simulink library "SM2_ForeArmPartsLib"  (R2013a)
settings: Solver=ode45  StartTime=0.0  StopTime=10.0  RelTol=1e-3
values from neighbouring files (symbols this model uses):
  ID = ID(val==max(val))    [PD_NarrowRange.m]    (also in NyquistMinDist_v1.m = find(D==minDist,1))
  m = v*BEAM.rho    [FlexBeamModelConstruct2.m]    (also in FlexBeamModelConstruct3.m = BEAM.rho*v; FlexBeam_1D_Construct.m = REF.m/REF.l*a.*(linspace(1-OPT.MassBiais+1e-6,1+OPT.MassBiai; FlexBeam_3D_Construct.m = REF.m/REF.l*a.*(linspace(1-OPT.MassBiais+1e-6,1+OPT.MassBiai; FreeFlexBeam_3D_Construct.m = REF.m/REF.l*a.*tmp2)
  N = D(1)+(H4^2+H3^2)/H2^2-(E(1)*H4+F(1)*H3)/H2    [MGD.m]    (also in MGD2.m)
  s = -sign(imag(KGZ_fr_tmp))    [LinprogReguliOptimFunc_1.m]    (also in LinprogReguliOptimFunc_2.m; LinprogReguliOptimFunc_1 - Copie.m)
  X = cos(phi(i))*x+sin(phi(i))*y    [MGI.m]
  Y = fft(y(:,i),NFFT)/L    [fft_bis.m]    (also in MGI.m = -sin(phi(i))*x+cos(phi(i))*y)
  Z = z    [MGI.m]
undefined symbols (not defined in the file or in its folder): kg, rad, SimParam
libraries: sm_lib x48, SM2_ForeArmPartsLib x42

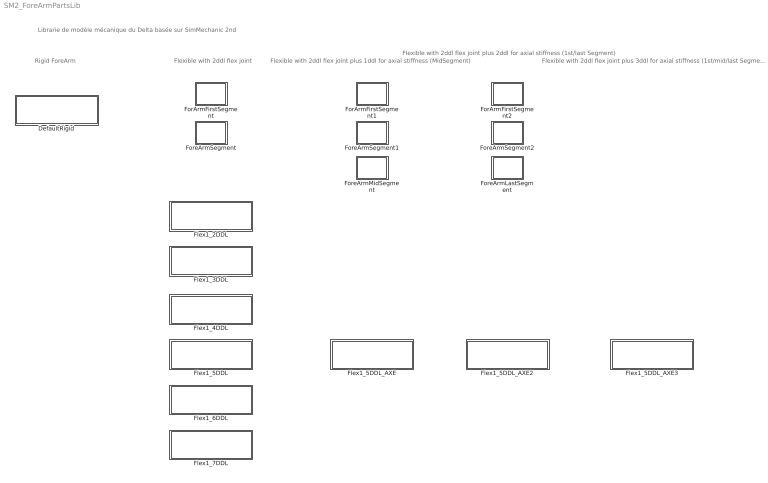
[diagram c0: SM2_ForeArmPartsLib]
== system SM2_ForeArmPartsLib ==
  note: Librarie de modèle mécanique du Delta basée sur SimMechanic 2nd
  note: Rigid ForeArm
  note: Flexible with 2ddl flex joint plus 1ddl for axial stiffness (MidSegment)
  note: Flexible with 2ddl flex joint
  note: Flexible with 2ddl flex joint plus 2ddl for axial stiffness (1st/last Segment)
  note: Flexible with 2ddl flex joint plus 3ddl for axial stiffness (1st/mid/last Segment)
  DefaultRigid : Subsystem  InitFcn=SimParam.ForeArm = RigidForeArm_paramInitFnc(RawParam,0);  VariantControl=foreArmVarDefault
  Flex1_2DDL : Subsystem  InitFcn=SimParam.ForeArm = flexPreCalcForeArm_paramInitFnc(RawParam,2);  VariantControl=foreArmVarFlex1_2ddl
  Flex1_3DDL : Subsystem  InitFcn=SimParam.ForeArm = flexPreCalcForeArm_paramInitFnc(RawParam,3);  VariantControl=foreArmVarFlex1_3ddl
  Flex1_4DDL : Subsystem  InitFcn=SimParam.ForeArm = flexPreCalcForeArm_paramInitFnc(RawParam,4);  VariantControl=foreArmVarFlex1_4ddl
  Flex1_5DDL : Subsystem  InitFcn=SimParam.ForeArm = flexPreCalcForeArm_paramInitFnc(RawParam,5);  VariantControl=foreArmVarFlex1_5ddl
  Flex1_5DDL_AXE : Subsystem  InitFcn=SimParam.ForeArm = flexPreCalcForeArm_paramInitFnc(RawParam,5,2);  VariantControl=foreArmVarFlex1_5ddl
  Flex1_5DDL_AXE2 : Subsystem  InitFcn=SimParam.ForeArm = flexPreCalcForeArm_paramInitFnc(RawParam,5,3);  VariantControl=foreArmVarFlex1_5ddl
  Flex1_5DDL_AXE3 : Subsystem  InitFcn=SimParam.ForeArm = flexPreCalcForeArm_paramInitFnc(RawParam,5,4);  VariantControl=foreArmVarFlex1_5ddl
  Flex1_6DDL : Subsystem  InitFcn=SimParam.ForeArm = flexPreCalcForeArm_paramInitFnc(RawParam,6);  VariantControl=foreArmVarFlex1_6ddl
  Flex1_7DDL : Subsystem  InitFcn=SimParam.ForeArm = flexPreCalcForeArm_paramInitFnc(RawParam,7);  VariantControl=foreArmVarFlex1_7ddl
  ForArmFirstSegment : Subsystem
  ForArmFirstSegment1 : Subsystem
  ForArmFirstSegment2 : Subsystem
  ForeArmLastSegment : Subsystem
  ForeArmMidSegment : Subsystem
  ForeArmSegment : Subsystem
  ForeArmSegment1 : Subsystem
  ForeArmSegment2 : Subsystem

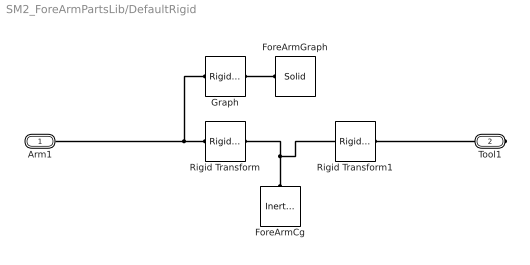
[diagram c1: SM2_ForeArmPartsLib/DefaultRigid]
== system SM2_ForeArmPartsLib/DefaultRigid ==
  ForeArmCg : sm_lib/Body Elements/Inertia  InertiaType=Custom  Mass=SimParam.ForeArm.m  MassUnits=kg  CenterOfMass=[0 0 0]  CenterOfMassUnits=m  MomentsOfInertia=SimParam.ForeArm.I  MomentsOfInertiaUnits=kg*m^2  ProductsOfInertia=[0 0 0]  ProductsOfInertiaUnits=kg*m^2  BlockFunction=simmechanics.library.body_elements.inertia
  ForeArmGraph : sm_lib/Body Elements/Solid  InertiaType=CalculateFromGeometry  Mass=0  MassUnits=kg  CenterOfMass=[0 0 0]  CenterOfMassUnits=m  MomentsOfInertia=[0 0 0]  MomentsOfInertiaUnits=kg*m^2  ProductsOfInertia=[0 0 0]  ProductsOfInertiaUnits=kg*m^2  DensityBased=on  Density=0  DensityUnits=kg/(m^3)  GraphicType=FromGeometry  MarkerShape=Sphere  MarkerSize=10  MarkerSizeUnits=m  GraphicVisPropType=SimpleVisualProperties  GraphicDiffuseColor=[0.5 0.5 0.5]  GraphicSpecularColor=[0.5 0.5 0.5 1.0]  GraphicAmbientColor=[0.15 0.15 0.15 1.0]  GraphicEmissiveColor=[0.0 0.0 0.0 1.0]  GraphicShininess=75  GraphicOpacity=1.0  GeometryShape=Cylinder  RectangleSize=[1 1]  RectangleSizeUnits=m  BrickDimensions=[0.3 0.02 0.02]  BrickDimensionUnits=m  CylinderRadius=5e-3  CylinderRadiusUnits=m  CylinderLength=SimParam.ForeArm.l  CylinderLengthUnits=m  SphereRadius=0.03  SphereRadiusUnits=m  EllipsoidRadii=[1 1 1]  EllipsoidRadiiUnits=m  ExtrusionCrossSection=1e-2.*[1 1; -1 1; -1 -1; 1 -1]  ExtrusionCrossSectionUnits=m  ExtrusionLength=SimParam.Arm.l  ExtrusionLengthUnits=m  PolygonNumSides=3  PolygonOuterRadius=1  PolygonOuterRadiusUnits=m  ExtGeomFileUnits=m  RevolutionCrossSection=[1 1; 1 -1; 2 -1; 2 1]  RevolutionCrossSectionUnits=m  RevolutionExtent=Full  RevolutionAngle=180  RevolutionAngleUnits=deg  BlockFunction=simmechanics.library.body_elements.solid
  Graph : sm_lib/Frames and  Transforms/Rigid  Transform  TranslationMethod=Cartesian  TranslationLengthUnit=m  TranslationStandardAxis=+Z  TranslationStandardOffset=0  TranslationCartesianOffset=[SimParam.ForeArm.l/2 0 0]  TranslationROffset=0  TranslationROffsetUnits=m  TranslationZOffset=0  TranslationZOffsetUnits=m  TranslationThetaOffset=0  TranslationThetaOffsetUnits=deg  RotationMethod=AlignedAxes  RotationAngleUnits=deg  RotationStandardAxis=+Z  RotationAngle=0  RotationArbitraryAxis=[0 0 1]  FollAlignAxisA=+Z  BaseAlignAxisA=+X  FollAlignAxisB=+Y  BaseAlignAxisB=+Z  BlockFunction=simmechanics.library.frames_transforms.rigid_transform
  Rigid Transform : sm_lib/Frames and  Transforms/Rigid  Transform  TranslationMethod=Cartesian  TranslationLengthUnit=m  TranslationStandardAxis=+Z  TranslationStandardOffset=0  TranslationCartesianOffset=[SimParam.ForeArm.lcg 0 0]  TranslationROffset=0  TranslationROffsetUnits=m  TranslationZOffset=0  TranslationZOffsetUnits=m  TranslationThetaOffset=0  TranslationThetaOffsetUnits=deg  RotationMethod=None  RotationAngleUnits=deg  RotationStandardAxis=+Z  RotationAngle=0  RotationArbitraryAxis=[0 0 1]  FollAlignAxisA=+X  BaseAlignAxisA=+Y  FollAlignAxisB=+Y  BaseAlignAxisB=+Z  BlockFunction=simmechanics.library.frames_transforms.rigid_transform
  Rigid Transform1 : sm_lib/Frames and  Transforms/Rigid  Transform  TranslationMethod=Cartesian  TranslationLengthUnit=m  TranslationStandardAxis=+Z  TranslationStandardOffset=0  TranslationCartesianOffset=[SimParam.ForeArm.l-SimParam.ForeArm.lcg 0 0]  TranslationROffset=0  TranslationROffsetUnits=m  TranslationZOffset=0  TranslationZOffsetUnits=m  TranslationThetaOffset=0  TranslationThetaOffsetUnits=deg  RotationMethod=AlignedAxes  RotationAngleUnits=deg  RotationStandardAxis=+Z  RotationAngle=0  RotationArbitraryAxis=[0 0 1]  FollAlignAxisA=-Z  BaseAlignAxisA=+X  FollAlignAxisB=+Y  BaseAlignAxisB=+Y  BlockFunction=simmechanics.library.frames_transforms.rigid_transform
  Arm1 : PMIOPort  Port=1  Side=Left
  Tool1 : PMIOPort  Port=2  Side=Right
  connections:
  ForeArmCg/RConn1 -- Rigid Transform/RConn1 -- Rigid Transform1/LConn1
  Graph/LConn1 -- Arm1/RConn1 -- Rigid Transform/LConn1
  Tool1/RConn1 -- Rigid Transform1/RConn1
  Graph/RConn1 -- ForeArmGraph/RConn1

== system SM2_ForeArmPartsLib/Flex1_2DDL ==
  ForArmFirstSegment : SM2_ForeArmPartsLib/ForArmFirstSegment  ID=1
  ForeArmSegment : SM2_ForeArmPartsLib/ForeArmSegment  ID=2
  Arm1 : PMIOPort  Port=1  Side=Left
  Tool1 : PMIOPort  Port=2  Side=Right
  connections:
  ForArmFirstSegment/LConn1 -- Arm1/RConn1
  ForArmFirstSegment/RConn1 -- ForeArmSegment/LConn1
  ForeArmSegment/RConn1 -- Tool1/RConn1

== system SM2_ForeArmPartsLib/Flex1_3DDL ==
  ForArmFirstSegment : SM2_ForeArmPartsLib/ForArmFirstSegment  ID=1
  ForeArmSegment : SM2_ForeArmPartsLib/ForeArmSegment  ID=2
  ForeArmSegment1 : SM2_ForeArmPartsLib/ForeArmSegment  ID=3
  Arm1 : PMIOPort  Port=1  Side=Left
  Tool1 : PMIOPort  Port=2  Side=Right
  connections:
  ForArmFirstSegment/LConn1 -- Arm1/RConn1
  ForArmFirstSegment/RConn1 -- ForeArmSegment/LConn1
  ForeArmSegment/RConn1 -- ForeArmSegment1/LConn1
  ForeArmSegment1/RConn1 -- Tool1/RConn1

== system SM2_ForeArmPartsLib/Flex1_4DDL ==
  ForArmFirstSegment : SM2_ForeArmPartsLib/ForArmFirstSegment  ID=1
  ForeArmSegment2 : SM2_ForeArmPartsLib/ForeArmSegment  ID=2
  ForeArmSegment3 : SM2_ForeArmPartsLib/ForeArmSegment  ID=3
  ForeArmSegment4 : SM2_ForeArmPartsLib/ForeArmSegment  ID=4
  Arm1 : PMIOPort  Port=1  Side=Left
  Tool1 : PMIOPort  Port=2  Side=Right
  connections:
  ForArmFirstSegment/LConn1 -- Arm1/RConn1
  ForArmFirstSegment/RConn1 -- ForeArmSegment2/LConn1
  ForeArmSegment2/RConn1 -- ForeArmSegment3/LConn1
  ForeArmSegment3/RConn1 -- ForeArmSegment4/LConn1
  ForeArmSegment4/RConn1 -- Tool1/RConn1

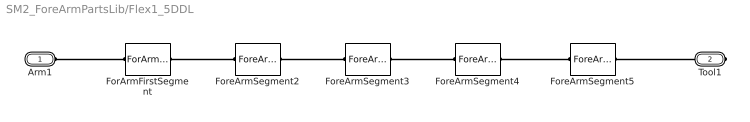
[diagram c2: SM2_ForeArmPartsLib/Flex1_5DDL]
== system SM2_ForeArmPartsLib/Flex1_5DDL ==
  ForArmFirstSegment : SM2_ForeArmPartsLib/ForArmFirstSegment  ID=1
  ForeArmSegment2 : SM2_ForeArmPartsLib/ForeArmSegment  ID=2
  ForeArmSegment3 : SM2_ForeArmPartsLib/ForeArmSegment  ID=3
  ForeArmSegment4 : SM2_ForeArmPartsLib/ForeArmSegment  ID=4
  ForeArmSegment5 : SM2_ForeArmPartsLib/ForeArmSegment  ID=5
  Arm1 : PMIOPort  Port=1  Side=Left
  Tool1 : PMIOPort  Port=2  Side=Right
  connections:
  ForArmFirstSegment/LConn1 -- Arm1/RConn1
  ForArmFirstSegment/RConn1 -- ForeArmSegment2/LConn1
  ForeArmSegment4/RConn1 -- ForeArmSegment5/LConn1
  ForeArmSegment4/LConn1 -- ForeArmSegment3/RConn1
  ForeArmSegment3/LConn1 -- ForeArmSegment2/RConn1
  ForeArmSegment5/RConn1 -- Tool1/RConn1

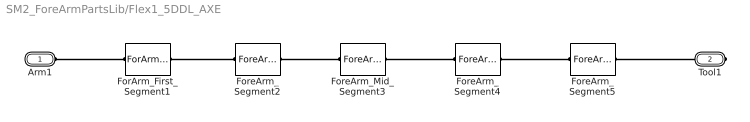
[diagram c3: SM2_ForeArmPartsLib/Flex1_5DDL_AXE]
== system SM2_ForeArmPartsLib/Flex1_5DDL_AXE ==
  ForArm_First_Segment1 : SM2_ForeArmPartsLib/ForArmFirstSegment1  ID=1
  ForeArm_Mid_Segment3 : SM2_ForeArmPartsLib/ForeArmMidSegment  ID=3
  ForeArm_Segment2 : SM2_ForeArmPartsLib/ForeArmSegment1  ID=2
  ForeArm_Segment4 : SM2_ForeArmPartsLib/ForeArmSegment1  ID=4
  ForeArm_Segment5 : SM2_ForeArmPartsLib/ForeArmSegment1  ID=5
  Arm1 : PMIOPort  Port=1  Side=Left
  Tool1 : PMIOPort  Port=2  Side=Right
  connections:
  ForArm_First_Segment1/LConn1 -- Arm1/RConn1
  ForeArm_Segment5/RConn1 -- Tool1/RConn1
  ForeArm_Segment5/LConn1 -- ForeArm_Segment4/RConn1
  ForeArm_Segment4/LConn1 -- ForeArm_Mid_Segment3/RConn1
  ForeArm_Mid_Segment3/LConn1 -- ForeArm_Segment2/RConn1
  ForeArm_Segment2/LConn1 -- ForArm_First_Segment1/RConn1

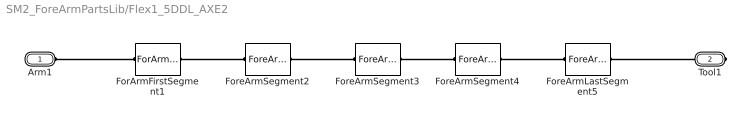
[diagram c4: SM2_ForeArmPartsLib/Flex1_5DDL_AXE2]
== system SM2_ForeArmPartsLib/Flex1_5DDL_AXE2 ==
  ForArmFirstSegment1 : SM2_ForeArmPartsLib/ForArmFirstSegment2  ID=1
  ForeArmLastSegment5 : SM2_ForeArmPartsLib/ForeArmLastSegment  ID=5
  ForeArmSegment2 : SM2_ForeArmPartsLib/ForeArmSegment2  ID=2
  ForeArmSegment3 : SM2_ForeArmPartsLib/ForeArmSegment2  ID=3
  ForeArmSegment4 : SM2_ForeArmPartsLib/ForeArmSegment2  ID=4
  Arm1 : PMIOPort  Port=1  Side=Left
  Tool1 : PMIOPort  Port=2  Side=Right
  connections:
  ForArmFirstSegment1/LConn1 -- Arm1/RConn1
  ForeArmLastSegment5/RConn1 -- Tool1/RConn1
  ForArmFirstSegment1/RConn1 -- ForeArmSegment2/LConn1
  ForeArmSegment2/RConn1 -- ForeArmSegment3/LConn1
  ForeArmSegment3/RConn1 -- ForeArmSegment4/LConn1
  ForeArmSegment4/RConn1 -- ForeArmLastSegment5/LConn1

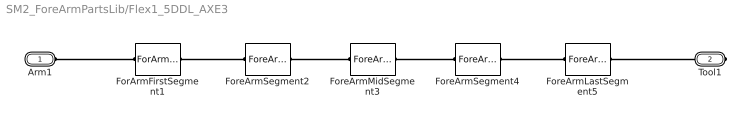
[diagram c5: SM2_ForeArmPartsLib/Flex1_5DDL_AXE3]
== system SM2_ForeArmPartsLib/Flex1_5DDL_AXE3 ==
  ForArmFirstSegment1 : SM2_ForeArmPartsLib/ForArmFirstSegment2  ID=1
  ForeArmLastSegment5 : SM2_ForeArmPartsLib/ForeArmLastSegment  ID=5
  ForeArmMidSegment3 : SM2_ForeArmPartsLib/ForeArmMidSegment  ID=3
  ForeArmSegment2 : SM2_ForeArmPartsLib/ForeArmSegment2  ID=2
  ForeArmSegment4 : SM2_ForeArmPartsLib/ForeArmSegment2  ID=4
  Arm1 : PMIOPort  Port=1  Side=Left
  Tool1 : PMIOPort  Port=2  Side=Right
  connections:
  ForArmFirstSegment1/LConn1 -- Arm1/RConn1
  ForeArmLastSegment5/RConn1 -- Tool1/RConn1
  ForArmFirstSegment1/RConn1 -- ForeArmSegment2/LConn1
  ForeArmSegment2/RConn1 -- ForeArmMidSegment3/LConn1
  ForeArmMidSegment3/RConn1 -- ForeArmSegment4/LConn1
  ForeArmSegment4/RConn1 -- ForeArmLastSegment5/LConn1

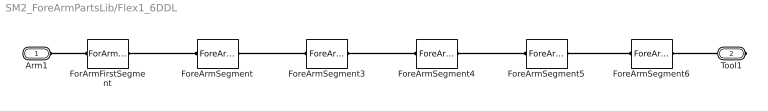
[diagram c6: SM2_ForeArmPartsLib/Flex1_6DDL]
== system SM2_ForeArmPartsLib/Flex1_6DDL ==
  ForArmFirstSegment : SM2_ForeArmPartsLib/ForArmFirstSegment  ID=1
  ForeArmSegment : SM2_ForeArmPartsLib/ForeArmSegment  ID=2
  ForeArmSegment3 : SM2_ForeArmPartsLib/ForeArmSegment  ID=3
  ForeArmSegment4 : SM2_ForeArmPartsLib/ForeArmSegment  ID=4
  ForeArmSegment5 : SM2_ForeArmPartsLib/ForeArmSegment  ID=5
  ForeArmSegment6 : SM2_ForeArmPartsLib/ForeArmSegment  ID=6
  Arm1 : PMIOPort  Port=1  Side=Left
  Tool1 : PMIOPort  Port=2  Side=Right
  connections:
  ForArmFirstSegment/LConn1 -- Arm1/RConn1
  ForeArmSegment6/RConn1 -- Tool1/RConn1
  ForArmFirstSegment/RConn1 -- ForeArmSegment/LConn1
  ForeArmSegment3/RConn1 -- ForeArmSegment4/LConn1
  ForeArmSegment4/RConn1 -- ForeArmSegment5/LConn1
  ForeArmSegment3/LConn1 -- ForeArmSegment/RConn1
  ForeArmSegment6/LConn1 -- ForeArmSegment5/RConn1

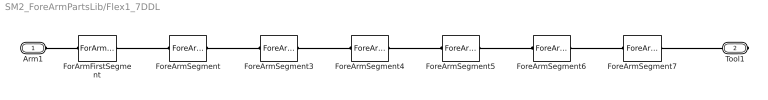
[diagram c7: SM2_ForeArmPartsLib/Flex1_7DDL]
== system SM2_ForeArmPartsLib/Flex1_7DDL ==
  ForArmFirstSegment : SM2_ForeArmPartsLib/ForArmFirstSegment  ID=1
  ForeArmSegment : SM2_ForeArmPartsLib/ForeArmSegment  ID=2
  ForeArmSegment3 : SM2_ForeArmPartsLib/ForeArmSegment  ID=3
  ForeArmSegment4 : SM2_ForeArmPartsLib/ForeArmSegment  ID=4
  ForeArmSegment5 : SM2_ForeArmPartsLib/ForeArmSegment  ID=5
  ForeArmSegment6 : SM2_ForeArmPartsLib/ForeArmSegment  ID=6
  ForeArmSegment7 : SM2_ForeArmPartsLib/ForeArmSegment  ID=7
  Arm1 : PMIOPort  Port=1  Side=Left
  Tool1 : PMIOPort  Port=2  Side=Right
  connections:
  ForArmFirstSegment/LConn1 -- Arm1/RConn1
  ForeArmSegment7/RConn1 -- Tool1/RConn1
  ForArmFirstSegment/RConn1 -- ForeArmSegment/LConn1
  ForeArmSegment7/LConn1 -- ForeArmSegment6/RConn1
  ForeArmSegment6/LConn1 -- ForeArmSegment5/RConn1
  ForeArmSegment5/LConn1 -- ForeArmSegment4/RConn1
  ForeArmSegment4/LConn1 -- ForeArmSegment3/RConn1
  ForeArmSegment3/LConn1 -- ForeArmSegment/RConn1

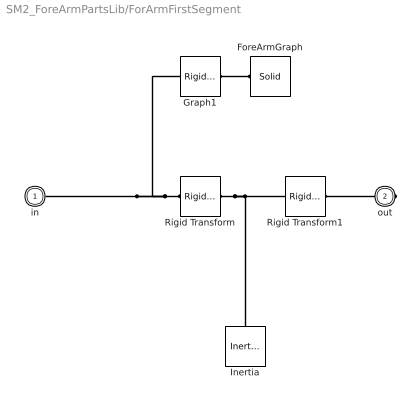
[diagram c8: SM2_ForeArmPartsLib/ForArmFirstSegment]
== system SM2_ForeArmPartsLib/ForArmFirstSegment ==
  ForeArmGraph : sm_lib/Body Elements/Solid  InertiaType=CalculateFromGeometry  Mass=0  MassUnits=kg  CenterOfMass=[0 0 0]  CenterOfMassUnits=m  MomentsOfInertia=[0 0 0]  MomentsOfInertiaUnits=kg*m^2  ProductsOfInertia=[0 0 0]  ProductsOfInertiaUnits=kg*m^2  DensityBased=on  Density=0  DensityUnits=kg/(m^3)  GraphicType=FromGeometry  MarkerShape=Sphere  MarkerSize=10  MarkerSizeUnits=m  GraphicVisPropType=SimpleVisualProperties  GraphicDiffuseColor=[0.5 0.5 0.5]  GraphicSpecularColor=[0.5 0.5 0.5 1.0]  GraphicAmbientColor=[0.15 0.15 0.15 1.0]  GraphicEmissiveColor=[0.0 0.0 0.0 1.0]  GraphicShininess=75  GraphicOpacity=1.0  GeometryShape=Cylinder  RectangleSize=[1 1]  RectangleSizeUnits=m  BrickDimensions=[0.3 0.02 0.02]  BrickDimensionUnits=m  CylinderRadius=5e-3  CylinderRadiusUnits=m  CylinderLength=SimParam.ForeArm.l(2,ID)  CylinderLengthUnits=m  SphereRadius=0.03  SphereRadiusUnits=m  EllipsoidRadii=[1 1 1]  EllipsoidRadiiUnits=m  ExtrusionCrossSection=1e-2.*[1 1; -1 1; -1 -1; 1 -1]  ExtrusionCrossSectionUnits=m  ExtrusionLength=SimParam.Arm.l  ExtrusionLengthUnits=m  PolygonNumSides=3  PolygonOuterRadius=1  PolygonOuterRadiusUnits=m  ExtGeomFileUnits=m  RevolutionCrossSection=[1 1; 1 -1; 2 -1; 2 1]  RevolutionCrossSectionUnits=m  RevolutionExtent=Full  RevolutionAngle=180  RevolutionAngleUnits=deg  BlockFunction=simmechanics.library.body_elements.solid
  Graph1 : sm_lib/Frames and  Transforms/Rigid  Transform  TranslationMethod=Cartesian  TranslationLengthUnit=m  TranslationStandardAxis=+Z  TranslationStandardOffset=0  TranslationCartesianOffset=[(SimParam.ForeArm.l(1,ID)+SimParam.ForeArm.l(2,ID))/2 0 0]  TranslationROffset=0  TranslationROffsetUnits=m  TranslationZOffset=0  TranslationZOffsetUnits=m  TranslationThetaOffset=0  TranslationThetaOffsetUnits=deg  RotationMethod=AlignedAxes  RotationAngleUnits=deg  RotationStandardAxis=+Z  RotationAngle=0  RotationArbitraryAxis=[0 0 1]  FollAlignAxisA=+Z  BaseAlignAxisA=+X  FollAlignAxisB=+Y  BaseAlignAxisB=+Z  BlockFunction=simmechanics.library.frames_transforms.rigid_transform
  Inertia : sm_lib/Body Elements/Inertia  InertiaType=Custom  Mass=SimParam.ForeArm.m(ID)  MassUnits=kg  CenterOfMass=[0 0 0]  CenterOfMassUnits=m  MomentsOfInertia=SimParam.ForeArm.I(:,ID)'  MomentsOfInertiaUnits=kg*m^2  ProductsOfInertia=[0 0 0]  ProductsOfInertiaUnits=kg*m^2  BlockFunction=simmechanics.library.body_elements.inertia
  Rigid Transform : sm_lib/Frames and  Transforms/Rigid  Transform  TranslationMethod=Cartesian  TranslationLengthUnit=m  TranslationStandardAxis=+Z  TranslationStandardOffset=0  TranslationCartesianOffset=[SimParam.ForeArm.l(1,ID) 0 0]  TranslationROffset=0  TranslationROffsetUnits=m  TranslationZOffset=0  TranslationZOffsetUnits=m  TranslationThetaOffset=0  TranslationThetaOffsetUnits=deg  RotationMethod=None  RotationAngleUnits=deg  RotationStandardAxis=+Z  RotationAngle=0  RotationArbitraryAxis=[0 0 1]  FollAlignAxisA=+X  BaseAlignAxisA=+Y  FollAlignAxisB=+Y  BaseAlignAxisB=+Z  BlockFunction=simmechanics.library.frames_transforms.rigid_transform
  Rigid Transform1 : sm_lib/Frames and  Transforms/Rigid  Transform  TranslationMethod=Cartesian  TranslationLengthUnit=m  TranslationStandardAxis=+Z  TranslationStandardOffset=0  TranslationCartesianOffset=[SimParam.ForeArm.l(2,ID) 0 0]  TranslationROffset=0  TranslationROffsetUnits=m  TranslationZOffset=0  TranslationZOffsetUnits=m  TranslationThetaOffset=0  TranslationThetaOffsetUnits=deg  RotationMethod=AlignedAxes  RotationAngleUnits=deg  RotationStandardAxis=+Z  RotationAngle=0  RotationArbitraryAxis=[0 0 1]  FollAlignAxisA=+Y  BaseAlignAxisA=+Y  FollAlignAxisB=-Z  BaseAlignAxisB=+X  BlockFunction=simmechanics.library.frames_transforms.rigid_transform
  in : PMIOPort  Port=1  Side=Left
  out : PMIOPort  Port=2  Side=Right
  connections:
  Rigid Transform/RConn1 -- Rigid Transform1/LConn1 -- Inertia/RConn1
  Rigid Transform/LConn1 -- in/RConn1 -- Graph1/LConn1
  Rigid Transform1/RConn1 -- out/RConn1
  Graph1/RConn1 -- ForeArmGraph/RConn1

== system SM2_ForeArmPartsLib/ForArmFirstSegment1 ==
  ForeArmGraph : sm_lib/Body Elements/Solid  InertiaType=CalculateFromGeometry  Mass=0  MassUnits=kg  CenterOfMass=[0 0 0]  CenterOfMassUnits=m  MomentsOfInertia=[0 0 0]  MomentsOfInertiaUnits=kg*m^2  ProductsOfInertia=[0 0 0]  ProductsOfInertiaUnits=kg*m^2  DensityBased=on  Density=0  DensityUnits=kg/(m^3)  GraphicType=FromGeometry  MarkerShape=Sphere  MarkerSize=10  MarkerSizeUnits=m  GraphicVisPropType=SimpleVisualProperties  GraphicDiffuseColor=[0.5 0.5 0.5]  GraphicSpecularColor=[0.5 0.5 0.5 1.0]  GraphicAmbientColor=[0.15 0.15 0.15 1.0]  GraphicEmissiveColor=[0.0 0.0 0.0 1.0]  GraphicShininess=75  GraphicOpacity=1.0  GeometryShape=Cylinder  RectangleSize=[1 1]  RectangleSizeUnits=m  BrickDimensions=[0.3 0.02 0.02]  BrickDimensionUnits=m  CylinderRadius=5e-3  CylinderRadiusUnits=m  CylinderLength=SimParam.ForeArm.l(2,ID)  CylinderLengthUnits=m  SphereRadius=0.03  SphereRadiusUnits=m  EllipsoidRadii=[1 1 1]  EllipsoidRadiiUnits=m  ExtrusionCrossSection=1e-2.*[1 1; -1 1; -1 -1; 1 -1]  ExtrusionCrossSectionUnits=m  ExtrusionLength=SimParam.Arm.l  ExtrusionLengthUnits=m  PolygonNumSides=3  PolygonOuterRadius=1  PolygonOuterRadiusUnits=m  ExtGeomFileUnits=m  RevolutionCrossSection=[1 1; 1 -1; 2 -1; 2 1]  RevolutionCrossSectionUnits=m  RevolutionExtent=Full  RevolutionAngle=180  RevolutionAngleUnits=deg  BlockFunction=simmechanics.library.body_elements.solid
  Graph1 : sm_lib/Frames and  Transforms/Rigid  Transform  TranslationMethod=Cartesian  TranslationLengthUnit=m  TranslationStandardAxis=+Z  TranslationStandardOffset=0  TranslationCartesianOffset=[(SimParam.ForeArm.l(1,ID)+SimParam.ForeArm.l(2,ID))/2 0 0]  TranslationROffset=0  TranslationROffsetUnits=m  TranslationZOffset=0  TranslationZOffsetUnits=m  TranslationThetaOffset=0  TranslationThetaOffsetUnits=deg  RotationMethod=AlignedAxes  RotationAngleUnits=deg  RotationStandardAxis=+Z  RotationAngle=0  RotationArbitraryAxis=[0 0 1]  FollAlignAxisA=+Z  BaseAlignAxisA=+X  FollAlignAxisB=+Y  BaseAlignAxisB=+Z  BlockFunction=simmechanics.library.frames_transforms.rigid_transform
  Inertia : sm_lib/Body Elements/Inertia  InertiaType=Custom  Mass=SimParam.ForeArm.m(ID)  MassUnits=kg  CenterOfMass=[0 0 0]  CenterOfMassUnits=m  MomentsOfInertia=SimParam.ForeArm.I(:,ID)'  MomentsOfInertiaUnits=kg*m^2  ProductsOfInertia=[0 0 0]  ProductsOfInertiaUnits=kg*m^2  BlockFunction=simmechanics.library.body_elements.inertia
  Rigid Transform : sm_lib/Frames and  Transforms/Rigid  Transform  TranslationMethod=Cartesian  TranslationLengthUnit=m  TranslationStandardAxis=+Z  TranslationStandardOffset=0  TranslationCartesianOffset=[SimParam.ForeArm.l(1,ID) 0 0]  TranslationROffset=0  TranslationROffsetUnits=m  TranslationZOffset=0  TranslationZOffsetUnits=m  TranslationThetaOffset=0  TranslationThetaOffsetUnits=deg  RotationMethod=None  RotationAngleUnits=deg  RotationStandardAxis=+Z  RotationAngle=0  RotationArbitraryAxis=[0 0 1]  FollAlignAxisA=+X  BaseAlignAxisA=+Y  FollAlignAxisB=+Y  BaseAlignAxisB=+Z  BlockFunction=simmechanics.library.frames_transforms.rigid_transform
  Rigid Transform1 : sm_lib/Frames and  Transforms/Rigid  Transform  TranslationMethod=Cartesian  TranslationLengthUnit=m  TranslationStandardAxis=+Z  TranslationStandardOffset=0  TranslationCartesianOffset=[SimParam.ForeArm.l(2,ID) 0 0]  TranslationROffset=0  TranslationROffsetUnits=m  TranslationZOffset=0  TranslationZOffsetUnits=m  TranslationThetaOffset=0  TranslationThetaOffsetUnits=deg  RotationMethod=AlignedAxes  RotationAngleUnits=deg  RotationStandardAxis=+Z  RotationAngle=0  RotationArbitraryAxis=[0 0 1]  FollAlignAxisA=+Y  BaseAlignAxisA=+Y  FollAlignAxisB=-Z  BaseAlignAxisB=+X  BlockFunction=simmechanics.library.frames_transforms.rigid_transform
  in : PMIOPort  Port=1  Side=Left
  out : PMIOPort  Port=2  Side=Right
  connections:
  Rigid Transform/RConn1 -- Rigid Transform1/LConn1 -- Inertia/RConn1
  Rigid Transform/LConn1 -- in/RConn1 -- Graph1/LConn1
  Rigid Transform1/RConn1 -- out/RConn1
  Graph1/RConn1 -- ForeArmGraph/RConn1

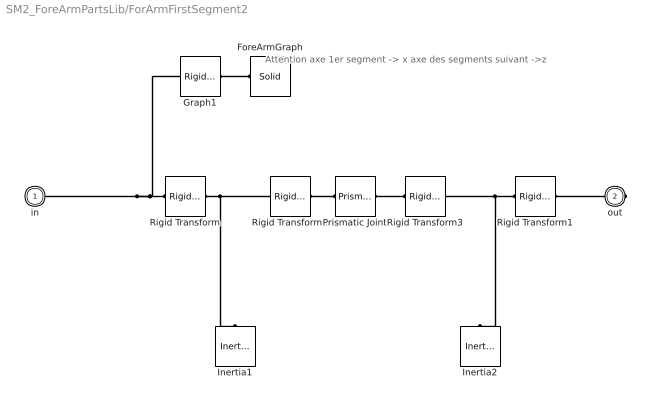
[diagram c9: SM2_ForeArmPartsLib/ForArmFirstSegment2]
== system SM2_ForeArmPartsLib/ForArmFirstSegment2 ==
  note: Attention axe 1er segment -> x axe des segments suivant ->z
  ForeArmGraph : sm_lib/Body Elements/Solid  InertiaType=CalculateFromGeometry  Mass=0  MassUnits=kg  CenterOfMass=[0 0 0]  CenterOfMassUnits=m  MomentsOfInertia=[0 0 0]  MomentsOfInertiaUnits=kg*m^2  ProductsOfInertia=[0 0 0]  ProductsOfInertiaUnits=kg*m^2  DensityBased=on  Density=0  DensityUnits=kg/(m^3)  GraphicType=FromGeometry  MarkerShape=Sphere  MarkerSize=10  MarkerSizeUnits=m  GraphicVisPropType=SimpleVisualProperties  GraphicDiffuseColor=[0.5 0.5 0.5]  GraphicSpecularColor=[0.5 0.5 0.5 1.0]  GraphicAmbientColor=[0.15 0.15 0.15 1.0]  GraphicEmissiveColor=[0.0 0.0 0.0 1.0]  GraphicShininess=75  GraphicOpacity=1.0  GeometryShape=Cylinder  RectangleSize=[1 1]  RectangleSizeUnits=m  BrickDimensions=[0.3 0.02 0.02]  BrickDimensionUnits=m  CylinderRadius=5e-3  CylinderRadiusUnits=m  CylinderLength=SimParam.ForeArm.l(2,ID)  CylinderLengthUnits=m  SphereRadius=0.03  SphereRadiusUnits=m  EllipsoidRadii=[1 1 1]  EllipsoidRadiiUnits=m  ExtrusionCrossSection=1e-2.*[1 1; -1 1; -1 -1; 1 -1]  ExtrusionCrossSectionUnits=m  ExtrusionLength=SimParam.Arm.l  ExtrusionLengthUnits=m  PolygonNumSides=3  PolygonOuterRadius=1  PolygonOuterRadiusUnits=m  ExtGeomFileUnits=m  RevolutionCrossSection=[1 1; 1 -1; 2 -1; 2 1]  RevolutionCrossSectionUnits=m  RevolutionExtent=Full  RevolutionAngle=180  RevolutionAngleUnits=deg  BlockFunction=simmechanics.library.body_elements.solid
  Graph1 : sm_lib/Frames and  Transforms/Rigid  Transform  TranslationMethod=Cartesian  TranslationLengthUnit=m  TranslationStandardAxis=+Z  TranslationStandardOffset=0  TranslationCartesianOffset=[(SimParam.ForeArm.l(1,ID)+SimParam.ForeArm.l(2,ID))/2 0 0]  TranslationROffset=0  TranslationROffsetUnits=m  TranslationZOffset=0  TranslationZOffsetUnits=m  TranslationThetaOffset=0  TranslationThetaOffsetUnits=deg  RotationMethod=AlignedAxes  RotationAngleUnits=deg  RotationStandardAxis=+Z  RotationAngle=0  RotationArbitraryAxis=[0 0 1]  FollAlignAxisA=+Z  BaseAlignAxisA=+X  FollAlignAxisB=+Y  BaseAlignAxisB=+Z  BlockFunction=simmechanics.library.frames_transforms.rigid_transform
  Inertia1 : sm_lib/Body Elements/Inertia  InertiaType=Custom  Mass=0.5*SimParam.ForeArm.m(ID)  MassUnits=kg  CenterOfMass=[0 0 0]  CenterOfMassUnits=m  MomentsOfInertia=0.5.*[SimParam.ForeArm.I(2:3,ID)',SimParam.ForeArm.I(1,ID)']  MomentsOfInertiaUnits=kg*m^2  ProductsOfInertia=[0 0 0]  ProductsOfInertiaUnits=kg*m^2  BlockFunction=simmechanics.library.body_elements.inertia
  Inertia2 : sm_lib/Body Elements/Inertia  InertiaType=Custom  Mass=0.5*SimParam.ForeArm.m(ID)  MassUnits=kg  CenterOfMass=[0 0 0]  CenterOfMassUnits=m  MomentsOfInertia=0.5.*[SimParam.ForeArm.I(2:3,ID)',SimParam.ForeArm.I(1,ID)']  MomentsOfInertiaUnits=kg*m^2  ProductsOfInertia=[0 0 0]  ProductsOfInertiaUnits=kg*m^2  BlockFunction=simmechanics.library.body_elements.inertia
  Prismatic Joint : sm_lib/Joints/Prismatic  Joint  SenseConstraintForceX=off  SenseConstraintForceY=off  SenseConstraintForceZ=off  SenseConstraintTorqueX=off  SenseConstraintTorqueY=off  SenseConstraintTorqueZ=off  ConstraintWrenchDir=FollowerOnBase  ConstraintWrenchFrame=BaseFrame  EquilibriumPosition=0  EquilibriumPositionUnits=m  SpringStiffness=SimParam.ForeArm.k(1,ID)  SpringStiffnessUnits=N/m  DampingCoefficient=SimParam.ForeArm.c(1,ID)  DampingCoefficientUnits=N/(m/s)  ActuationMode=NoActuation  SensePosition=off  SenseVelocity=off  SenseAcceleration=off  SenseTorqueForce=off  PositionTargetValue=0  PositionTargetValueUnits=m  PositionTargetSpecify=on  PositionTargetPriority=High  VelocityTargetValue=0  VelocityTargetValueUnits=m/s  VelocityTargetSpecify=on  VelocityTargetPriority=High  BlockFunction=simmechanics.library.joints.prismatic_joint
  Rigid Transform : sm_lib/Frames and  Transforms/Rigid  Transform  TranslationMethod=Cartesian  TranslationLengthUnit=m  TranslationStandardAxis=+Z  TranslationStandardOffset=0  TranslationCartesianOffset=[SimParam.ForeArm.l(1,ID) 0 0]  TranslationROffset=0  TranslationROffsetUnits=m  TranslationZOffset=0  TranslationZOffsetUnits=m  TranslationThetaOffset=0  TranslationThetaOffsetUnits=deg  RotationMethod=None  RotationAngleUnits=deg  RotationStandardAxis=+Z  RotationAngle=0  RotationArbitraryAxis=[0 0 1]  FollAlignAxisA=+X  BaseAlignAxisA=+Y  FollAlignAxisB=+Y  BaseAlignAxisB=+Z  BlockFunction=simmechanics.library.frames_transforms.rigid_transform
  Rigid Transform1 : sm_lib/Frames and  Transforms/Rigid  Transform  TranslationMethod=Cartesian  TranslationLengthUnit=m  TranslationStandardAxis=+Z  TranslationStandardOffset=0  TranslationCartesianOffset=[SimParam.ForeArm.l(2,ID) 0 0]  TranslationROffset=0  TranslationROffsetUnits=m  TranslationZOffset=0  TranslationZOffsetUnits=m  TranslationThetaOffset=0  TranslationThetaOffsetUnits=deg  RotationMethod=AlignedAxes  RotationAngleUnits=deg  RotationStandardAxis=+Z  RotationAngle=0  RotationArbitraryAxis=[0 0 1]  FollAlignAxisA=+Y  BaseAlignAxisA=+Y  FollAlignAxisB=-Z  BaseAlignAxisB=+X  BlockFunction=simmechanics.library.frames_transforms.rigid_transform
  Rigid Transform2 : sm_lib/Frames and  Transforms/Rigid  Transform  TranslationMethod=None  TranslationLengthUnit=m  TranslationStandardAxis=+Z  TranslationStandardOffset=0  TranslationCartesianOffset=[0 0 0]  TranslationROffset=0  TranslationROffsetUnits=m  TranslationZOffset=0  TranslationZOffsetUnits=m  TranslationThetaOffset=0  TranslationThetaOffsetUnits=deg  RotationMethod=AlignedAxes  RotationAngleUnits=deg  RotationStandardAxis=+Z  RotationAngle=0  RotationArbitraryAxis=[0 0 1]  FollAlignAxisA=+Z  BaseAlignAxisA=+X  FollAlignAxisB=+Y  BaseAlignAxisB=+Y  BlockFunction=simmechanics.library.frames_transforms.rigid_transform
  Rigid Transform3 : sm_lib/Frames and  Transforms/Rigid  Transform  TranslationMethod=None  TranslationLengthUnit=m  TranslationStandardAxis=+Z  TranslationStandardOffset=0  TranslationCartesianOffset=[0 0 0]  TranslationROffset=0  TranslationROffsetUnits=m  TranslationZOffset=0  TranslationZOffsetUnits=m  TranslationThetaOffset=0  TranslationThetaOffsetUnits=deg  RotationMethod=AlignedAxes  RotationAngleUnits=deg  RotationStandardAxis=+Z  RotationAngle=0  RotationArbitraryAxis=[0 0 1]  FollAlignAxisA=+X  BaseAlignAxisA=+Z  FollAlignAxisB=+Y  BaseAlignAxisB=+Y  BlockFunction=simmechanics.library.frames_transforms.rigid_transform
  in : PMIOPort  Port=1  Side=Left
  out : PMIOPort  Port=2  Side=Right
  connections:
  Rigid Transform/LConn1 -- in/RConn1 -- Graph1/LConn1
  Rigid Transform1/RConn1 -- out/RConn1
  Graph1/RConn1 -- ForeArmGraph/RConn1
  Rigid Transform/RConn1 -- Rigid Transform2/LConn1 -- Inertia1/RConn1
  Rigid Transform1/LConn1 -- Rigid Transform3/RConn1 -- Inertia2/RConn1
  Prismatic Joint/LConn1 -- Rigid Transform2/RConn1
  Rigid Transform3/LConn1 -- Prismatic Joint/RConn1

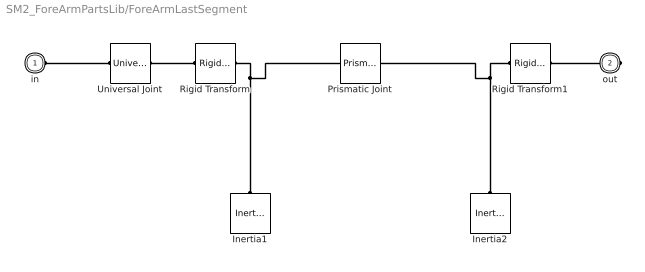
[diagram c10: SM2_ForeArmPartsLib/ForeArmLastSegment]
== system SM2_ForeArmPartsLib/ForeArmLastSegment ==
  Inertia1 : sm_lib/Body Elements/Inertia  InertiaType=Custom  Mass=0.5*SimParam.ForeArm.m(ID)  MassUnits=kg  CenterOfMass=[0 0 0]  CenterOfMassUnits=m  MomentsOfInertia=0.5.*[SimParam.ForeArm.I(2:3,ID)',SimParam.ForeArm.I(1,ID)']  MomentsOfInertiaUnits=kg*m^2  ProductsOfInertia=[0 0 0]  ProductsOfInertiaUnits=kg*m^2  BlockFunction=simmechanics.library.body_elements.inertia
  Inertia2 : sm_lib/Body Elements/Inertia  InertiaType=Custom  Mass=0.5*SimParam.ForeArm.m(ID)  MassUnits=kg  CenterOfMass=[0 0 0]  CenterOfMassUnits=m  MomentsOfInertia=0.5.*[SimParam.ForeArm.I(2:3,ID)',SimParam.ForeArm.I(1,ID)']  MomentsOfInertiaUnits=kg*m^2  ProductsOfInertia=[0 0 0]  ProductsOfInertiaUnits=kg*m^2  BlockFunction=simmechanics.library.body_elements.inertia
  Prismatic Joint : sm_lib/Joints/Prismatic  Joint  SenseConstraintForceX=off  SenseConstraintForceY=off  SenseConstraintForceZ=off  SenseConstraintTorqueX=off  SenseConstraintTorqueY=off  SenseConstraintTorqueZ=off  ConstraintWrenchDir=FollowerOnBase  ConstraintWrenchFrame=BaseFrame  EquilibriumPosition=0  EquilibriumPositionUnits=m  SpringStiffness=SimParam.ForeArm.k(1,ID)  SpringStiffnessUnits=N/m  DampingCoefficient=SimParam.ForeArm.c(1,ID)  DampingCoefficientUnits=N/(m/s)  ActuationMode=NoActuation  SensePosition=off  SenseVelocity=off  SenseAcceleration=off  SenseTorqueForce=off  PositionTargetValue=0  PositionTargetValueUnits=m  PositionTargetSpecify=on  PositionTargetPriority=High  VelocityTargetValue=0  VelocityTargetValueUnits=m/s  VelocityTargetSpecify=on  VelocityTargetPriority=High  BlockFunction=simmechanics.library.joints.prismatic_joint
  Rigid Transform : sm_lib/Frames and  Transforms/Rigid  Transform  TranslationMethod=Cartesian  TranslationLengthUnit=m  TranslationStandardAxis=+Z  TranslationStandardOffset=0  TranslationCartesianOffset=[0 0 -SimParam.ForeArm.l(1,ID)]  TranslationROffset=0  TranslationROffsetUnits=m  TranslationZOffset=0  TranslationZOffsetUnits=m  TranslationThetaOffset=0  TranslationThetaOffsetUnits=deg  RotationMethod=None  RotationAngleUnits=deg  RotationStandardAxis=+Z  RotationAngle=0  RotationArbitraryAxis=[0 0 1]  FollAlignAxisA=+Y  BaseAlignAxisA=+Y  FollAlignAxisB=+X  BaseAlignAxisB=-Z  BlockFunction=simmechanics.library.frames_transforms.rigid_transform
  Rigid Transform1 : sm_lib/Frames and  Transforms/Rigid  Transform  TranslationMethod=Cartesian  TranslationLengthUnit=m  TranslationStandardAxis=+Z  TranslationStandardOffset=0  TranslationCartesianOffset=[0 0 -SimParam.ForeArm.l(2,ID)]  TranslationROffset=0  TranslationROffsetUnits=m  TranslationZOffset=0  TranslationZOffsetUnits=m  TranslationThetaOffset=0  TranslationThetaOffsetUnits=deg  RotationMethod=None  RotationAngleUnits=deg  RotationStandardAxis=+Z  RotationAngle=0  RotationArbitraryAxis=[0 0 1]  FollAlignAxisA=+Y  BaseAlignAxisA=+Y  FollAlignAxisB=-Z  BaseAlignAxisB=+X  BlockFunction=simmechanics.library.frames_transforms.rigid_transform
  Universal Joint : sm_lib/Joints/Universal  Joint  SenseConstraintForceX=off  SenseConstraintForceY=off  SenseConstraintForceZ=off  SenseConstraintTorqueX=off  SenseConstraintTorqueY=off  SenseConstraintTorqueZ=off  ConstraintWrenchDir=FollowerOnBase  ConstraintWrenchFrame=BaseFrame  RxEquilibriumPosition=0  RxEquilibriumPositionUnits=rad  RxSpringStiffness=SimParam.ForeArm.k(6,ID)  RxSpringStiffnessUnits=N*m/rad  RxDampingCoefficient=SimParam.ForeArm.c(6,ID)  RxDampingCoefficientUnits=N*m/(rad/s)  RxActuationMode=NoActuation  RxSensePosition=off  RxSenseVelocity=off  RxSenseAcceleration=off  RxSenseTorqueForce=off  RxPositionTargetValue=0  RxPositionTargetValueUnits=rad  RxPositionTargetSpecify=on  RxPositionTargetPriority=Low  RxVelocityTargetValue=0  RxVelocityTargetValueUnits=rad/s  RxVelocityTargetSpecify=on  RxVelocityTargetPriority=High  RyEquilibriumPosition=0  RyEquilibriumPositionUnits=rad  RySpringStiffness=SimParam.ForeArm.k(5,ID)  RySpringStiffnessUnits=N*m/rad  RyDampingCoefficient=SimParam.ForeArm.c(5,ID)  RyDampingCoefficientUnits=N*m/(rad/s)  RyActuationMode=NoActuation  RySensePosition=off  RySenseVelocity=off  RySenseAcceleration=off  RySenseTorqueForce=off  RyPositionTargetValue=0  RyPositionTargetValueUnits=rad  RyPositionTargetSpecify=on  RyPositionTargetPriority=Low  RyVelocityTargetValue=0  RyVelocityTargetValueUnits=rad/s  RyVelocityTargetSpecify=on  RyVelocityTargetPriority=High  BlockFunction=simmechanics.library.joints.universal_joint
  in : PMIOPort  Port=1  Side=Left
  out : PMIOPort  Port=2  Side=Right
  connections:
  Universal Joint/RConn1 -- Rigid Transform/LConn1
  Rigid Transform1/RConn1 -- out/RConn1
  Universal Joint/LConn1 -- in/RConn1
  Inertia1/RConn1 -- Prismatic Joint/LConn1 -- Rigid Transform/RConn1
  Inertia2/RConn1 -- Prismatic Joint/RConn1 -- Rigid Transform1/LConn1

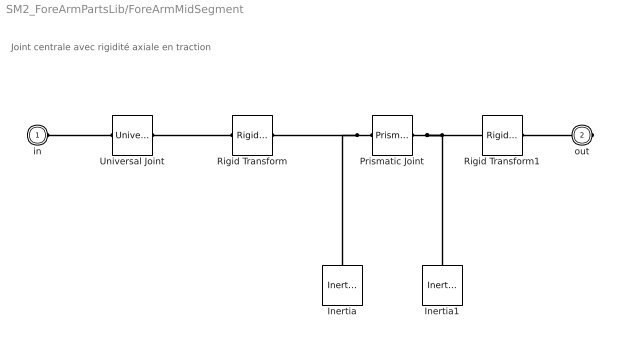
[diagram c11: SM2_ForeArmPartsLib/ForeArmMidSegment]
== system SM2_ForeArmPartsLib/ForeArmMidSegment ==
  note: Joint centrale avec rigidité axiale en traction
  Inertia : sm_lib/Body Elements/Inertia  InertiaType=Custom  Mass=0.5*SimParam.ForeArm.m(ID)  MassUnits=kg  CenterOfMass=[0 0 0]  CenterOfMassUnits=m  MomentsOfInertia=0.5.*[SimParam.ForeArm.I(2:3,ID)',SimParam.ForeArm.I(1,ID)']  MomentsOfInertiaUnits=kg*m^2  ProductsOfInertia=[0 0 0]  ProductsOfInertiaUnits=kg*m^2  BlockFunction=simmechanics.library.body_elements.inertia
  Inertia1 : sm_lib/Body Elements/Inertia  InertiaType=Custom  Mass=0.5*SimParam.ForeArm.m(ID)  MassUnits=kg  CenterOfMass=[0 0 0]  CenterOfMassUnits=m  MomentsOfInertia=0.5.*[SimParam.ForeArm.I(2:3,ID)',SimParam.ForeArm.I(1,ID)']  MomentsOfInertiaUnits=kg*m^2  ProductsOfInertia=[0 0 0]  ProductsOfInertiaUnits=kg*m^2  BlockFunction=simmechanics.library.body_elements.inertia
  Prismatic Joint : sm_lib/Joints/Prismatic  Joint  SenseConstraintForceX=off  SenseConstraintForceY=off  SenseConstraintForceZ=off  SenseConstraintTorqueX=off  SenseConstraintTorqueY=off  SenseConstraintTorqueZ=off  ConstraintWrenchDir=FollowerOnBase  ConstraintWrenchFrame=BaseFrame  EquilibriumPosition=0  EquilibriumPositionUnits=m  SpringStiffness=SimParam.ForeArm.k(1,ID)  SpringStiffnessUnits=N/m  DampingCoefficient=SimParam.ForeArm.c(1,ID)  DampingCoefficientUnits=N/(m/s)  ActuationMode=NoActuation  SensePosition=off  SenseVelocity=off  SenseAcceleration=off  SenseTorqueForce=off  PositionTargetValue=0  PositionTargetValueUnits=m  PositionTargetSpecify=on  PositionTargetPriority=High  VelocityTargetValue=0  VelocityTargetValueUnits=m/s  VelocityTargetSpecify=on  VelocityTargetPriority=High  BlockFunction=simmechanics.library.joints.prismatic_joint
  Rigid Transform : sm_lib/Frames and  Transforms/Rigid  Transform  TranslationMethod=Cartesian  TranslationLengthUnit=m  TranslationStandardAxis=+Z  TranslationStandardOffset=0  TranslationCartesianOffset=[0 0 -SimParam.ForeArm.l(1,ID)]  TranslationROffset=0  TranslationROffsetUnits=m  TranslationZOffset=0  TranslationZOffsetUnits=m  TranslationThetaOffset=0  TranslationThetaOffsetUnits=deg  RotationMethod=None  RotationAngleUnits=deg  RotationStandardAxis=+Z  RotationAngle=0  RotationArbitraryAxis=[0 0 1]  FollAlignAxisA=+Y  BaseAlignAxisA=+Y  FollAlignAxisB=+X  BaseAlignAxisB=-Z  BlockFunction=simmechanics.library.frames_transforms.rigid_transform
  Rigid Transform1 : sm_lib/Frames and  Transforms/Rigid  Transform  TranslationMethod=Cartesian  TranslationLengthUnit=m  TranslationStandardAxis=+Z  TranslationStandardOffset=0  TranslationCartesianOffset=[0 0 -SimParam.ForeArm.l(2,ID)]  TranslationROffset=0  TranslationROffsetUnits=m  TranslationZOffset=0  TranslationZOffsetUnits=m  TranslationThetaOffset=0  TranslationThetaOffsetUnits=deg  RotationMethod=None  RotationAngleUnits=deg  RotationStandardAxis=+Z  RotationAngle=0  RotationArbitraryAxis=[0 0 1]  FollAlignAxisA=+Y  BaseAlignAxisA=+Y  FollAlignAxisB=-Z  BaseAlignAxisB=+X  BlockFunction=simmechanics.library.frames_transforms.rigid_transform
  Universal Joint : sm_lib/Joints/Universal  Joint  SenseConstraintForceX=off  SenseConstraintForceY=off  SenseConstraintForceZ=off  SenseConstraintTorqueX=off  SenseConstraintTorqueY=off  SenseConstraintTorqueZ=off  ConstraintWrenchDir=FollowerOnBase  ConstraintWrenchFrame=BaseFrame  RxEquilibriumPosition=0  RxEquilibriumPositionUnits=rad  RxSpringStiffness=SimParam.ForeArm.k(6,ID)  RxSpringStiffnessUnits=N*m/rad  RxDampingCoefficient=SimParam.ForeArm.c(6,ID)  RxDampingCoefficientUnits=N*m/(rad/s)  RxActuationMode=NoActuation  RxSensePosition=off  RxSenseVelocity=off  RxSenseAcceleration=off  RxSenseTorqueForce=off  RxPositionTargetValue=0  RxPositionTargetValueUnits=rad  RxPositionTargetSpecify=on  RxPositionTargetPriority=Low  RxVelocityTargetValue=0  RxVelocityTargetValueUnits=rad/s  RxVelocityTargetSpecify=on  RxVelocityTargetPriority=High  RyEquilibriumPosition=0  RyEquilibriumPositionUnits=rad  RySpringStiffness=SimParam.ForeArm.k(5,ID)  RySpringStiffnessUnits=N*m/rad  RyDampingCoefficient=SimParam.ForeArm.c(5,ID)  RyDampingCoefficientUnits=N*m/(rad/s)  RyActuationMode=NoActuation  RySensePosition=off  RySenseVelocity=off  RySenseAcceleration=off  RySenseTorqueForce=off  RyPositionTargetValue=0  RyPositionTargetValueUnits=rad  RyPositionTargetSpecify=on  RyPositionTargetPriority=Low  RyVelocityTargetValue=0  RyVelocityTargetValueUnits=rad/s  RyVelocityTargetSpecify=on  RyVelocityTargetPriority=High  BlockFunction=simmechanics.library.joints.universal_joint
  in : PMIOPort  Port=1  Side=Left
  out : PMIOPort  Port=2  Side=Right
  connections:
  Universal Joint/RConn1 -- Rigid Transform/LConn1
  Rigid Transform1/RConn1 -- out/RConn1
  Universal Joint/LConn1 -- in/RConn1
  Prismatic Joint/LConn1 -- Inertia/RConn1 -- Rigid Transform/RConn1
  Prismatic Joint/RConn1 -- Inertia1/RConn1 -- Rigid Transform1/LConn1

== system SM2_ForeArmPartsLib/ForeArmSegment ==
  Inertia : sm_lib/Body Elements/Inertia  InertiaType=Custom  Mass=SimParam.ForeArm.m(ID)  MassUnits=kg  CenterOfMass=[0 0 0]  CenterOfMassUnits=m  MomentsOfInertia=[SimParam.ForeArm.I(2:3,ID)',SimParam.ForeArm.I(1,ID)']  MomentsOfInertiaUnits=kg*m^2  ProductsOfInertia=[0 0 0]  ProductsOfInertiaUnits=kg*m^2  BlockFunction=simmechanics.library.body_elements.inertia
  Rigid Transform : sm_lib/Frames and  Transforms/Rigid  Transform  TranslationMethod=Cartesian  TranslationLengthUnit=m  TranslationStandardAxis=+Z  TranslationStandardOffset=0  TranslationCartesianOffset=[0 0 -SimParam.ForeArm.l(1,ID)]  TranslationROffset=0  TranslationROffsetUnits=m  TranslationZOffset=0  TranslationZOffsetUnits=m  TranslationThetaOffset=0  TranslationThetaOffsetUnits=deg  RotationMethod=None  RotationAngleUnits=deg  RotationStandardAxis=+Z  RotationAngle=0  RotationArbitraryAxis=[0 0 1]  FollAlignAxisA=+Y  BaseAlignAxisA=+Y  FollAlignAxisB=+X  BaseAlignAxisB=-Z  BlockFunction=simmechanics.library.frames_transforms.rigid_transform
  Rigid Transform1 : sm_lib/Frames and  Transforms/Rigid  Transform  TranslationMethod=Cartesian  TranslationLengthUnit=m  TranslationStandardAxis=+Z  TranslationStandardOffset=0  TranslationCartesianOffset=[0 0 -SimParam.ForeArm.l(2,ID)]  TranslationROffset=0  TranslationROffsetUnits=m  TranslationZOffset=0  TranslationZOffsetUnits=m  TranslationThetaOffset=0  TranslationThetaOffsetUnits=deg  RotationMethod=None  RotationAngleUnits=deg  RotationStandardAxis=+Z  RotationAngle=0  RotationArbitraryAxis=[0 0 1]  FollAlignAxisA=+Y  BaseAlignAxisA=+Y  FollAlignAxisB=-Z  BaseAlignAxisB=+X  BlockFunction=simmechanics.library.frames_transforms.rigid_transform
  Universal Joint : sm_lib/Joints/Universal  Joint  SenseConstraintForceX=off  SenseConstraintForceY=off  SenseConstraintForceZ=off  SenseConstraintTorqueX=off  SenseConstraintTorqueY=off  SenseConstraintTorqueZ=off  ConstraintWrenchDir=FollowerOnBase  ConstraintWrenchFrame=BaseFrame  RxEquilibriumPosition=0  RxEquilibriumPositionUnits=rad  RxSpringStiffness=SimParam.ForeArm.k(3,ID)  RxSpringStiffnessUnits=N*m/rad  RxDampingCoefficient=SimParam.ForeArm.c(3,ID)  RxDampingCoefficientUnits=N*m/(rad/s)  RxActuationMode=NoActuation  RxSensePosition=off  RxSenseVelocity=off  RxSenseAcceleration=off  RxSenseTorqueForce=off  RxPositionTargetValue=0  RxPositionTargetValueUnits=rad  RxPositionTargetSpecify=on  RxPositionTargetPriority=High  RxVelocityTargetValue=0  RxVelocityTargetValueUnits=rad/s  RxVelocityTargetSpecify=on  RxVelocityTargetPriority=High  RyEquilibriumPosition=0  RyEquilibriumPositionUnits=rad  RySpringStiffness=SimParam.ForeArm.k(2,ID)  RySpringStiffnessUnits=N*m/rad  RyDampingCoefficient=SimParam.ForeArm.c(2,ID)  RyDampingCoefficientUnits=N*m/(rad/s)  RyActuationMode=NoActuation  RySensePosition=off  RySenseVelocity=off  RySenseAcceleration=off  RySenseTorqueForce=off  RyPositionTargetValue=0  RyPositionTargetValueUnits=rad  RyPositionTargetSpecify=on  RyPositionTargetPriority=High  RyVelocityTargetValue=0  RyVelocityTargetValueUnits=rad/s  RyVelocityTargetSpecify=on  RyVelocityTargetPriority=High  BlockFunction=simmechanics.library.joints.universal_joint
  in : PMIOPort  Port=1  Side=Left
  out : PMIOPort  Port=2  Side=Right
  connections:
  Rigid Transform/RConn1 -- Inertia/RConn1 -- Rigid Transform1/LConn1
  Universal Joint/RConn1 -- Rigid Transform/LConn1
  Rigid Transform1/RConn1 -- out/RConn1
  Universal Joint/LConn1 -- in/RConn1

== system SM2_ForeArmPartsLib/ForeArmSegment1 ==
  Inertia : sm_lib/Body Elements/Inertia  InertiaType=Custom  Mass=SimParam.ForeArm.m(ID)  MassUnits=kg  CenterOfMass=[0 0 0]  CenterOfMassUnits=m  MomentsOfInertia=[SimParam.ForeArm.I(2:3,ID)',SimParam.ForeArm.I(1,ID)']  MomentsOfInertiaUnits=kg*m^2  ProductsOfInertia=[0 0 0]  ProductsOfInertiaUnits=kg*m^2  BlockFunction=simmechanics.library.body_elements.inertia
  Rigid Transform : sm_lib/Frames and  Transforms/Rigid  Transform  TranslationMethod=Cartesian  TranslationLengthUnit=m  TranslationStandardAxis=+Z  TranslationStandardOffset=0  TranslationCartesianOffset=[0 0 -SimParam.ForeArm.l(1,ID)]  TranslationROffset=0  TranslationROffsetUnits=m  TranslationZOffset=0  TranslationZOffsetUnits=m  TranslationThetaOffset=0  TranslationThetaOffsetUnits=deg  RotationMethod=None  RotationAngleUnits=deg  RotationStandardAxis=+Z  RotationAngle=0  RotationArbitraryAxis=[0 0 1]  FollAlignAxisA=+Y  BaseAlignAxisA=+Y  FollAlignAxisB=+X  BaseAlignAxisB=-Z  BlockFunction=simmechanics.library.frames_transforms.rigid_transform
  Rigid Transform1 : sm_lib/Frames and  Transforms/Rigid  Transform  TranslationMethod=Cartesian  TranslationLengthUnit=m  TranslationStandardAxis=+Z  TranslationStandardOffset=0  TranslationCartesianOffset=[0 0 -SimParam.ForeArm.l(2,ID)]  TranslationROffset=0  TranslationROffsetUnits=m  TranslationZOffset=0  TranslationZOffsetUnits=m  TranslationThetaOffset=0  TranslationThetaOffsetUnits=deg  RotationMethod=None  RotationAngleUnits=deg  RotationStandardAxis=+Z  RotationAngle=0  RotationArbitraryAxis=[0 0 1]  FollAlignAxisA=+Y  BaseAlignAxisA=+Y  FollAlignAxisB=-Z  BaseAlignAxisB=+X  BlockFunction=simmechanics.library.frames_transforms.rigid_transform
  Universal Joint : sm_lib/Joints/Universal  Joint  SenseConstraintForceX=off  SenseConstraintForceY=off  SenseConstraintForceZ=off  SenseConstraintTorqueX=off  SenseConstraintTorqueY=off  SenseConstraintTorqueZ=off  ConstraintWrenchDir=FollowerOnBase  ConstraintWrenchFrame=BaseFrame  RxEquilibriumPosition=0  RxEquilibriumPositionUnits=rad  RxSpringStiffness=SimParam.ForeArm.k(6,ID)  RxSpringStiffnessUnits=N*m/rad  RxDampingCoefficient=SimParam.ForeArm.c(6,ID)  RxDampingCoefficientUnits=N*m/(rad/s)  RxActuationMode=NoActuation  RxSensePosition=off  RxSenseVelocity=off  RxSenseAcceleration=off  RxSenseTorqueForce=off  RxPositionTargetValue=0  RxPositionTargetValueUnits=rad  RxPositionTargetSpecify=on  RxPositionTargetPriority=Low  RxVelocityTargetValue=0  RxVelocityTargetValueUnits=rad/s  RxVelocityTargetSpecify=on  RxVelocityTargetPriority=High  RyEquilibriumPosition=0  RyEquilibriumPositionUnits=rad  RySpringStiffness=SimParam.ForeArm.k(5,ID)  RySpringStiffnessUnits=N*m/rad  RyDampingCoefficient=SimParam.ForeArm.c(5,ID)  RyDampingCoefficientUnits=N*m/(rad/s)  RyActuationMode=NoActuation  RySensePosition=off  RySenseVelocity=off  RySenseAcceleration=off  RySenseTorqueForce=off  RyPositionTargetValue=0  RyPositionTargetValueUnits=rad  RyPositionTargetSpecify=on  RyPositionTargetPriority=Low  RyVelocityTargetValue=0  RyVelocityTargetValueUnits=rad/s  RyVelocityTargetSpecify=on  RyVelocityTargetPriority=High  BlockFunction=simmechanics.library.joints.universal_joint
  in : PMIOPort  Port=1  Side=Left
  out : PMIOPort  Port=2  Side=Right
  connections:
  Rigid Transform/RConn1 -- Inertia/RConn1 -- Rigid Transform1/LConn1
  Universal Joint/RConn1 -- Rigid Transform/LConn1
  Rigid Transform1/RConn1 -- out/RConn1
  Universal Joint/LConn1 -- in/RConn1

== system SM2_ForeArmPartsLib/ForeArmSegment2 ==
  Inertia : sm_lib/Body Elements/Inertia  InertiaType=Custom  Mass=SimParam.ForeArm.m(ID)  MassUnits=kg  CenterOfMass=[0 0 0]  CenterOfMassUnits=m  MomentsOfInertia=[SimParam.ForeArm.I(2:3,ID)',SimParam.ForeArm.I(1,ID)']  MomentsOfInertiaUnits=kg*m^2  ProductsOfInertia=[0 0 0]  ProductsOfInertiaUnits=kg*m^2  BlockFunction=simmechanics.library.body_elements.inertia
  Rigid Transform : sm_lib/Frames and  Transforms/Rigid  Transform  TranslationMethod=Cartesian  TranslationLengthUnit=m  TranslationStandardAxis=+Z  TranslationStandardOffset=0  TranslationCartesianOffset=[0 0 -SimParam.ForeArm.l(1,ID)]  TranslationROffset=0  TranslationROffsetUnits=m  TranslationZOffset=0  TranslationZOffsetUnits=m  TranslationThetaOffset=0  TranslationThetaOffsetUnits=deg  RotationMethod=None  RotationAngleUnits=deg  RotationStandardAxis=+Z  RotationAngle=0  RotationArbitraryAxis=[0 0 1]  FollAlignAxisA=+Y  BaseAlignAxisA=+Y  FollAlignAxisB=+X  BaseAlignAxisB=-Z  BlockFunction=simmechanics.library.frames_transforms.rigid_transform
  Rigid Transform1 : sm_lib/Frames and  Transforms/Rigid  Transform  TranslationMethod=Cartesian  TranslationLengthUnit=m  TranslationStandardAxis=+Z  TranslationStandardOffset=0  TranslationCartesianOffset=[0 0 -SimParam.ForeArm.l(2,ID)]  TranslationROffset=0  TranslationROffsetUnits=m  TranslationZOffset=0  TranslationZOffsetUnits=m  TranslationThetaOffset=0  TranslationThetaOffsetUnits=deg  RotationMethod=None  RotationAngleUnits=deg  RotationStandardAxis=+Z  RotationAngle=0  RotationArbitraryAxis=[0 0 1]  FollAlignAxisA=+Y  BaseAlignAxisA=+Y  FollAlignAxisB=-Z  BaseAlignAxisB=+X  BlockFunction=simmechanics.library.frames_transforms.rigid_transform
  Universal Joint : sm_lib/Joints/Universal  Joint  SenseConstraintForceX=off  SenseConstraintForceY=off  SenseConstraintForceZ=off  SenseConstraintTorqueX=off  SenseConstraintTorqueY=off  SenseConstraintTorqueZ=off  ConstraintWrenchDir=FollowerOnBase  ConstraintWrenchFrame=BaseFrame  RxEquilibriumPosition=0  RxEquilibriumPositionUnits=rad  RxSpringStiffness=SimParam.ForeArm.k(6,ID)  RxSpringStiffnessUnits=N*m/rad  RxDampingCoefficient=SimParam.ForeArm.c(6,ID)  RxDampingCoefficientUnits=N*m/(rad/s)  RxActuationMode=NoActuation  RxSensePosition=off  RxSenseVelocity=off  RxSenseAcceleration=off  RxSenseTorqueForce=off  RxPositionTargetValue=0  RxPositionTargetValueUnits=rad  RxPositionTargetSpecify=on  RxPositionTargetPriority=Low  RxVelocityTargetValue=0  RxVelocityTargetValueUnits=rad/s  RxVelocityTargetSpecify=on  RxVelocityTargetPriority=High  RyEquilibriumPosition=0  RyEquilibriumPositionUnits=rad  RySpringStiffness=SimParam.ForeArm.k(5,ID)  RySpringStiffnessUnits=N*m/rad  RyDampingCoefficient=SimParam.ForeArm.c(5,ID)  RyDampingCoefficientUnits=N*m/(rad/s)  RyActuationMode=NoActuation  RySensePosition=off  RySenseVelocity=off  RySenseAcceleration=off  RySenseTorqueForce=off  RyPositionTargetValue=0  RyPositionTargetValueUnits=rad  RyPositionTargetSpecify=on  RyPositionTargetPriority=Low  RyVelocityTargetValue=0  RyVelocityTargetValueUnits=rad/s  RyVelocityTargetSpecify=on  RyVelocityTargetPriority=High  BlockFunction=simmechanics.library.joints.universal_joint
  in : PMIOPort  Port=1  Side=Left
  out : PMIOPort  Port=2  Side=Right
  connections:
  Rigid Transform/RConn1 -- Inertia/RConn1 -- Rigid Transform1/LConn1
  Universal Joint/RConn1 -- Rigid Transform/LConn1
  Rigid Transform1/RConn1 -- out/RConn1
  Universal Joint/LConn1 -- in/RConn1
